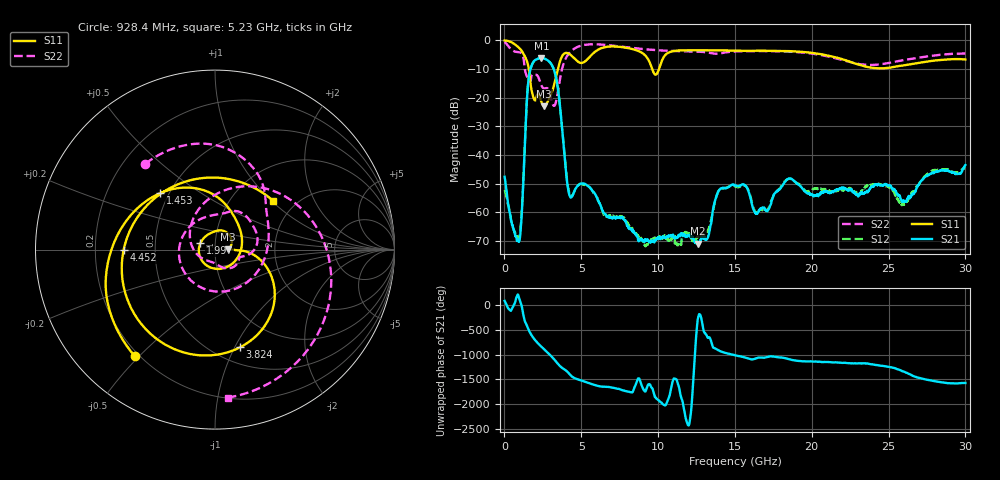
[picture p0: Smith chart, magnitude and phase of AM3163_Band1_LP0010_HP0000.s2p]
!Agilent Technologies,E8364B,MY43040894,A.07.50.67
!Agilent E8364B: A.07.50.67
!Date: Thursday, August 20, 2020 11:23:41
!Correction: S11(Full 2 Port(1,2))
!S21(Full 2 Port(1,2))
!S12(Full 2 Port(1,2))
!S22(Full 2 Port(1,2))
!S2P File: Measurements: S11, S21, S12, S22:
# Hz S  dB  R 50
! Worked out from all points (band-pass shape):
!   3201 points, 10 MHz to 30 GHz, reference 50 ohm
!   highest |S21| = -6.25 dB at 2.4 GHz (marker M1); lowest = -70.9 dB at 12.62 GHz (marker M2)
!   |S21| within 3 dB of the highest: 1.743 GHz to 3.142 GHz (1.399 GHz wide, 57.3 % of centre)
!   lowest |S11| = -23.1 dB at 2.587 GHz (marker M3), VSWR 1.15, Z = 57.6 + j0.102 ohm
!   |S11| at or under -10 dB: 1.584 GHz to 3.482 GHz (1.897 GHz wide, 74.9 % of centre); 9.611 GHz to 10.06 GHz (448.5 MHz wide, 4.56 % of centre)
!   |S22| runs from -22.9 to -0.6 dB; largest |S21 - S12| = 0.0063
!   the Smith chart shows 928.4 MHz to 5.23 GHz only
!   S11 on the Smith chart (normalised r, x): 928.4 MHz: 0.18, -0.49; 1.453 GHz: 0.45, +0.35; 1.997 GHz: 0.85, +0.06; 3.824 GHz: 0.66, -1.05; 4.452 GHz: 0.33, -0.00; 5.23 GHz: 1.55, +1.02
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1e7  -0.11 -8.9  -47.59 86.5  -52.25 -54.6  -0.62 -27.5
4.785938e8  -0.81 -63.7  -63.86 -80.3  -63.70 -100.6  -3.44 -149.2
9.284438e8  -2.58 -126.9  -70.19 171.3  -68.85 -70.7  -4.21 129.1
1.453269e9  -7.17 134.0  -21.44 -48.4  -21.43 -48.2  -12.53 -83.2
1.996838e9  -21.03 156.4  -6.95 13.5  -6.95 13.5  -12.05 31.0
2.399828e9  -21.60 7.3  -6.25 -117.6  -6.25 -117.6  -15.70 -13.1
2.587266e9  -23.06 0.7  -6.42 -172.7  -6.43 -172.8  -16.89 -18.1
2.905909e9  -20.35 0.1  -7.43 93.9  -7.45 93.8  -17.85 -54.9
3.318272e9  -13.66 -6.6  -12.07 -43.7  -12.09 -43.6  -22.18 -131.4
3.824353e9  -5.01 -75.5  -35.11 158.8  -35.06 158.3  -8.59 69.8
4.452269e9  -5.87 -179.8  -53.97 -14.2  -53.89 -14.8  -3.32 -18.8
5.014581e9  -7.95 79.7  -49.94 -83.1  -50.18 -85.9  -1.88 -68.9
5.230134e9  -7.47 39.9  -50.08 -106.5  -50.49 -107.1  -1.64 -84.9
6.364131e9  -2.70 -98.5  -59.22 154.2  -59.31 153.9  -1.56 -152.5
7.516872e9  -2.35 -175.9  -61.75 102.5  -61.33 106.1  -2.22 154.9
1.000979e10  -10.75 112.0  -69.08 -119.0  -68.80 117.0  -3.54 59.2
1.261517e10  -3.52 -0.3  -70.90 122.2  -68.51 94.8  -4.03 -29.3
1.5005e10  -3.64 -72.1  -50.58 66.5  -50.92 69.3  -3.93 -90.3
2.000958e10  -4.42 163.4  -53.82 -57.1  -52.27 -60.5  -4.68 136.8
2.276491e10  -8.05 59.9  -53.21 -93.8  -52.64 -106.3  -8.01 21.2
2.500479e10  -9.64 -62.1  -50.51 -164.5  -51.02 -165.9  -7.98 -92.2
3e10  -6.75 104.6  -43.51 -130.9  -44.63 -133.5  -4.64 103.0
